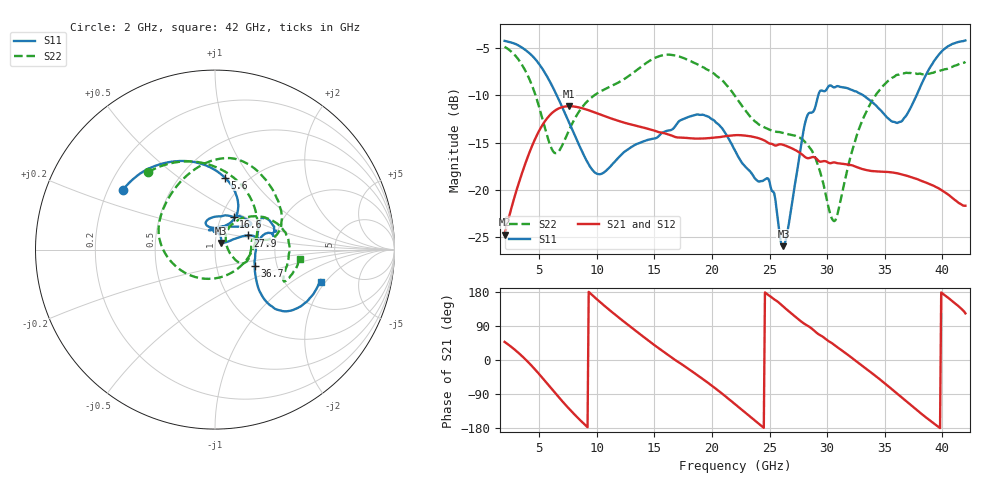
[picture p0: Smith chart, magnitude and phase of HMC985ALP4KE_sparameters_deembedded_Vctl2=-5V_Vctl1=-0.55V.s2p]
!s2p File: Measurements: S11, S21, S12, S22
# GHz S dB R 50.0
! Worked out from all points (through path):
!   401 points, 2 GHz to 42 GHz, reference 50 ohm
!   highest |S21| = -11.16 dB at 7.6 GHz (marker M1); lowest = -24.7 dB at 2 GHz (marker M2)
!   lowest |S11| = -25.9 dB at 26.2 GHz (marker M3), VSWR 1.11, Z = 53.5 + j3.9 ohm
!   |S11| at or under -10 dB: 6.522 GHz to 29.23 GHz (22.71 GHz wide, 127 % of centre); 33.11 GHz to 37.77 GHz (4.652 GHz wide, 13.1 % of centre)
!   |S22| runs from -23.3 to -4.9 dB; largest |S21 - S12| = 0.00029
!   S11 on the Smith chart (normalised r, x): 2 GHz: 0.26, +0.27; 5.6 GHz: 0.79, +0.76; 16.6 GHz: 1.14, +0.44; 27.9 GHz: 1.42, +0.23; 36.7 GHz: 1.54, -0.30; 42 GHz: 3.09, -1.78
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2  -4.26 147.3  -24.75 47.8  -24.76 47.8  -4.88 130.8
3.6  -5.05 120.7  -17.91 7.7  -17.92 7.8  -6.98 85.6
5.6  -7.85 82.2  -12.58 -58.7  -12.59 -58.6  -13.89 -4.9
6.5  -9.94 67.5  -11.53 -91.1  -11.53 -91.1  -16.11 -73.9
7.6  -12.87 58.1  -11.16 -128.8  -11.17 -128.8  -13.68 -139.6
8.7  -15.89 62.3  -11.37 -162.9  -11.37 -162.9  -11.32 -172.8
10.1  -18.32 87.6  -11.94 157.9  -11.95 157.9  -9.76 164.6
11.9  -16.58 109.6  -12.72 112.2  -12.73 112.3  -8.65 140.3
15.4  -14.30 77.2  -13.91 30.6  -13.91 30.6  -5.89 86.7
16.6  -13.57 60.2  -14.32 4.1  -14.32 4.1  -5.76 72.3
19.5  -12.19 34.9  -14.56 -56.6  -14.56 -56.6  -7.25 33.9
22  -15.84 52.5  -14.22 -116.5  -14.24 -116.5  -10.07 10.9
24.9  -18.83 100.9  -15.04 171.3  -15.05 171.3  -13.60 12.5
26.2  -25.95 46.1  -15.25 140.8  -15.25 140.8  -13.99 -2.1
27.9  -14.08 23.5  -16.35 98.0  -16.35 98.1  -14.71 -23.3
28.7  -11.83 11.7  -16.54 82.0  -16.55 82.0  -15.91 -27.8
30.7  -9.15 19.6  -17.11 37.8  -17.12 37.8  -23.24 24.3
32.9  -9.86 33.0  -17.74 -12.1  -17.75 -12.1  -13.12 50.5
35.4  -12.55 10.6  -18.12 -71.6  -18.13 -71.6  -8.40 21.2
36.7  -12.39 -22.3  -18.44 -104.6  -18.45 -104.6  -7.68 5.1
39.6  -5.87 -42.4  -19.79 -175.3  -19.79 -175.2  -7.51 -24.6
42  -4.22 -16.9  -21.68 123.1  -21.68 123.1  -6.47 -6.2
